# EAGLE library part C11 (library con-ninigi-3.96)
NINIGI
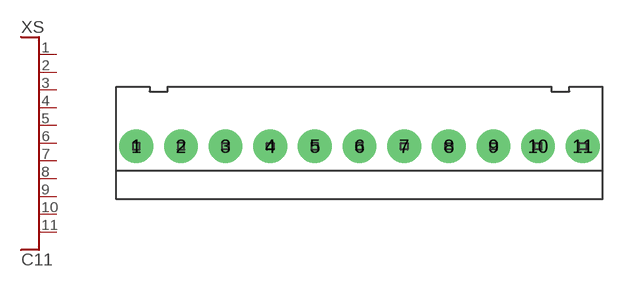
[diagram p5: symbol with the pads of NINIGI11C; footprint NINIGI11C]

Designator prefix XS

## C11  [NINIGI11C]
1  P$1
2  P$2
3  P$3
4  P$4
5  P$5
6  P$6
7  P$7
8  P$8
9  P$9
10  P$10
11  P$11

## Footprint NINIGI11C (pad centres in mm)
drill 1.6 pad 3: 1 -19.8,0; 2 -15.84,0; 3 -11.88,0; 4 -7.92,0; 5 -3.96,0; 6 0,0; 7 3.96,0; 8 7.92,0; 9 11.88,0; 10 15.84,0; 11 19.8,0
